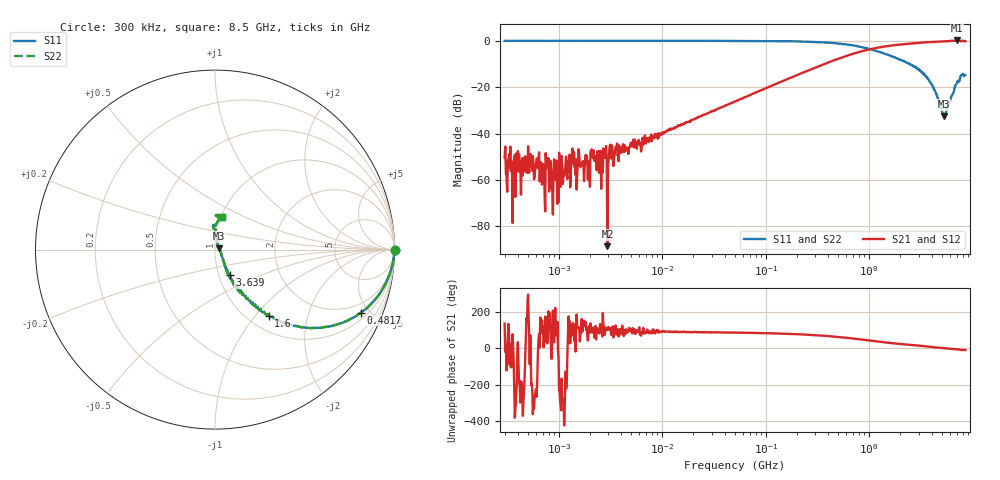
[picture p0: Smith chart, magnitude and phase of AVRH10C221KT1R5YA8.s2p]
! S-Parameter Data Generated by TDK Corporation
! Copyright(C) 2023 TDK Corporation.
! All Rights Reserved.
! TDK P/N: AVRH10C221KT1R5YA8 (Varistor)
! Property: V1mA=220V
! Size(LxWxT): 1x0.5x0.5mm
! Model Type: s2p (Touchstone File Format Version 1.0)
! Frequency: DC=Yes Start=0.3MHz Stop=8500MHz 802points Log-sweep
! Model Generated on Oct. 12, 2023
! Port Assignments:
!  1 ---N--- 2
! Applicable Conditions:
!  Temperature = 25 degC
!  DC Bias Voltage = 0 V
!  Small Signal Operation
! Terms and conditions regarding TDK Simulation Models
! (1)This simulation model is being provided solely for informational purposes. Please refer to the specifications of the products in terms of detailed characteristics of such products.
! (2)In no event shall TDK Corporation of any of its subsidiaries be liable for any loss or damage arising, directly or indirectly,
!  From any information contained in this simulation model, including, but not limited to loss or damages arising from any inaccuracies, omissions or errors in connection with such information.
! (3)Any and all copyrights on this simulation model are owned by TDK Corporation.
!  Duplication or redistribution of this simulation model without prior written permission from TDK Corporation is prohibited.
! (4)This simulation model is subject to any modification or change without any prior notice.
! (5)Neither TDK Corporation nor any of its subsidiaries shall make any warranty, express or implied,
!  Including but not limited to the correctness, implied warranties of merchantability and fitness for a particular purpose with respect to this simulation models.
! (6)The use of this simulation model shall be deemed to have consented to the terms and conditions hereof.
# Hz S MA R 50
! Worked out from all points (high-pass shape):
!   801 points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, 300 kHz to 8.5 GHz, reference 50 ohm
!   highest |S21| = 0.17 dB at 7.093 GHz (marker M1); lowest = -88.6 dB at 2.952 MHz (marker M2)
!   |S21| within 3 dB of the highest: 1.249 GHz to end of sweep
!   lowest |S11| = -32.6 dB at 5.285 GHz (marker M3), VSWR 1.05, Z = 52.3 + j0.697 ohm
!   |S11| at or under -10 dB: 2.446 GHz to end of sweep
!   |S22| runs from -32.6 to 0.0 dB; largest |S21 - S12| = 0
!   S11 on the Smith chart (normalised r, x): 300 kHz: open; 481.7 MHz: 1.36, -4.43; 1.6 GHz: 1.24, -1.18; 3.639 GHz: 1.13, -0.33; 8.5 GHz: 1.01, +0.38
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300000  1.002 -0.1  0.003067 134.0  0.003067 134.0  1.002 -0.1
363016  0.9981 0.0  0.001898 -4.2  0.001898 -4.2  0.9981 0.0
403527  0.9965 -0.1  0.004188 32.6  0.004188 32.6  0.9965 -0.1
637705  0.998 -0.1  0.00285 46.4  0.00285 46.4  0.998 -0.1
706047  1.001 -0.1  0.002227 118.8  0.002227 118.8  1.001 -0.1
784376  0.9983 -0.1  0.002645 51.3  0.002645 51.3  0.9983 -0.1
854988  0.9996 0.0  0.0007088 -59.1  0.0007088 -59.1  0.9996 0.0
1372418  1.003 -0.2  0.00398 137.4  0.00398 137.4  1.003 -0.2
1667335  1.002 -0.0  0.002131 159.6  0.002131 159.6  1.002 -0.0
2143129  1.001 -0.2  0.00296 109.8  0.00296 109.8  1.001 -0.2
2952450  1 -0.0  3.73e-05 112.0  3.73e-05 112.0  1 -0.0
3164401  1.002 -0.3  0.005748 109.2  0.005748 109.2  1.002 -0.3
9160262  0.999 -0.6  0.01012 84.3  0.01012 84.3  0.999 -0.6
5.049752e7  0.9971 -2.8  0.04937 85.2  0.04937 85.2  0.9971 -2.8
2.804659e8  0.953 -14.3  0.2483 72.0  0.2483 72.0  0.953 -14.3
4.816988e8  0.8854 -23.4  0.398 61.9  0.398 61.9  0.8854 -23.4
1.542892e9  0.4937 -49.3  0.7747 28.9  0.7747 28.9  0.4937 -49.3
1.599581e9  0.4751 -50.9  0.7914 27.8  0.7914 27.8  0.4751 -50.9
3.638769e9  0.1622 -59.9  0.9293 8.7  0.9293 8.7  0.1622 -59.9
5.285154e9  0.02355 16.4  0.9774 -0.4  0.9774 -0.4  0.02355 16.4
7.09348e9  0.1308 95.2  1.02 -7.3  1.02 -7.3  0.1308 95.2
8.5e9  0.1842 77.6  0.9772 -10.6  0.9772 -10.6  0.1842 77.6
